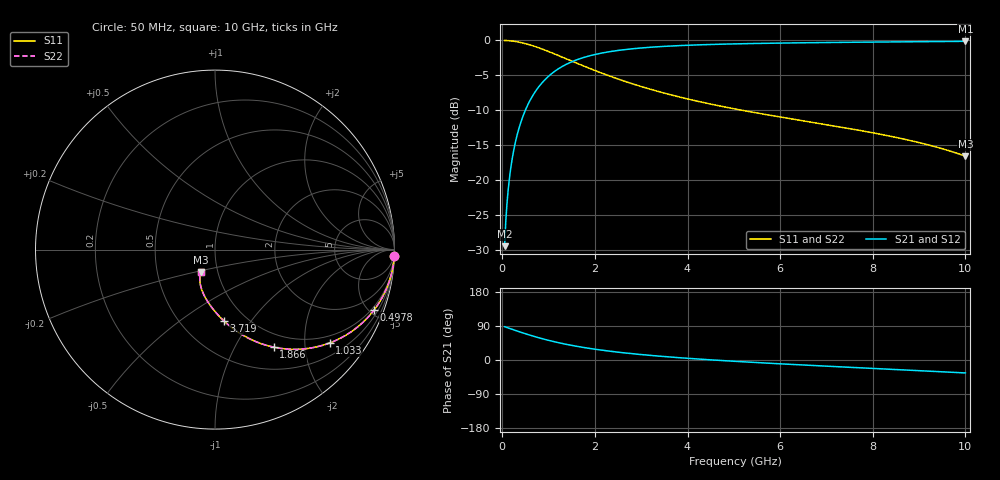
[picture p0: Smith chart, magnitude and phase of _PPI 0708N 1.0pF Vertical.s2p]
! S-Parameter data specifications (vertical orientation):
! Substrate: 40-mil Rogers 3003C, Substrate thickness, H=1.016mm, Dielectric constant, Er=3, Conductor thickness, T_mtl=0.043mm, Loss Tangent, Tand=0.003
! PCB Mounting Pad Footprint: Pad width, PadW=2.54mm , Pad length, PadL=0.51mm , Pad gap, PadG (edge-to-edge)=0.71mm , Reference planes=1.73mm apart
! Created Tue Jan 16 08:42:03 2018
# GHz S MA R 50
! 2 Port Network Data from SP1.SP block
! freq  magS11  angS11  magS21  angS21  magS12  angS12  magS22  angS22
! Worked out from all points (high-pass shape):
!   801 points, 50 MHz to 10 GHz, reference 50 ohm
!   highest |S21| = -0.13 dB at 10 GHz (marker M1); lowest = -29.5 dB at 50 MHz (marker M2)
!   |S21| within 3 dB of the highest: 1.477 GHz to end of sweep
!   lowest |S11| = -16.6 dB at 10 GHz (marker M3), VSWR 1.35, Z = 41.4 - j10.5 ohm
!   |S11| at or under -10 dB: 5.164 GHz to end of sweep
!   |S22| runs from -16.6 to 0.0 dB; largest |S21 - S12| = 0
!   S11 on the Smith chart (normalised r, x): 50 MHz: 1, -53; 497.8 MHz: 0.80, -5.37; 1.033 GHz: 0.80, -2.60; 1.866 GHz: 0.80, -1.45; 3.719 GHz: 0.79, -0.75; 10 GHz: 0.83, -0.21
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0.05  0.9994 -2.1  0.0335 87.9  0.0335 87.9  0.9994 -2.1
0.074875  0.9987 -3.2  0.05012 86.8  0.05012 86.8  0.9987 -3.2
0.124625  0.9965 -5.3  0.08324 84.7  0.08324 84.7  0.9965 -5.3
0.1495  0.995 -6.4  0.09969 83.6  0.09969 83.6  0.995 -6.4
0.1868125  0.9922 -8.0  0.1242 82.0  0.1242 82.0  0.9922 -8.0
0.224125  0.9889 -9.6  0.1485 80.4  0.1485 80.4  0.9889 -9.6
0.2863125  0.9821 -12.2  0.1884 77.8  0.1884 77.8  0.9821 -12.2
0.3485  0.9738 -14.7  0.2273 75.3  0.2273 75.3  0.9738 -14.7
0.49775  0.9487 -20.7  0.3159 69.3  0.3159 69.3  0.9487 -20.7
0.7340625  0.8978 -29.4  0.44 60.6  0.44 60.6  0.8978 -29.4
1.032563  0.8242 -39.1  0.5658 50.8  0.5658 50.8  0.8242 -39.1
1.3435  0.7472 -47.7  0.6639 42.3  0.6639 42.3  0.7472 -47.7
1.716625  0.6637 -56.1  0.7472 33.8  0.7472 33.8  0.6637 -56.1
1.865875  0.6337 -59.0  0.7727 30.9  0.7727 30.9  0.6337 -59.0
2.18925  0.576 -64.6  0.8165 25.3  0.8165 25.3  0.576 -64.6
2.5375  0.5235 -69.7  0.8509 20.1  0.8509 20.1  0.5235 -69.7
3.370812  0.4302 -79.5  0.9014 10.4  0.9014 10.4  0.4302 -79.5
3.719063  0.401 -82.8  0.9146 7.0  0.9146 7.0  0.401 -82.8
5.025  0.3226 -93.2  0.9447 -3.5  0.9447 -3.5  0.3226 -93.2
6.691625  0.2588 -104.0  0.9636 -14.4  0.9636 -14.4  0.2588 -104.0
8.345812  0.2068 -113.5  0.9755 -24.2  0.9755 -24.2  0.2068 -113.5
10  0.148 -122.8  0.9852 -34.2  0.9852 -34.2  0.148 -122.8
